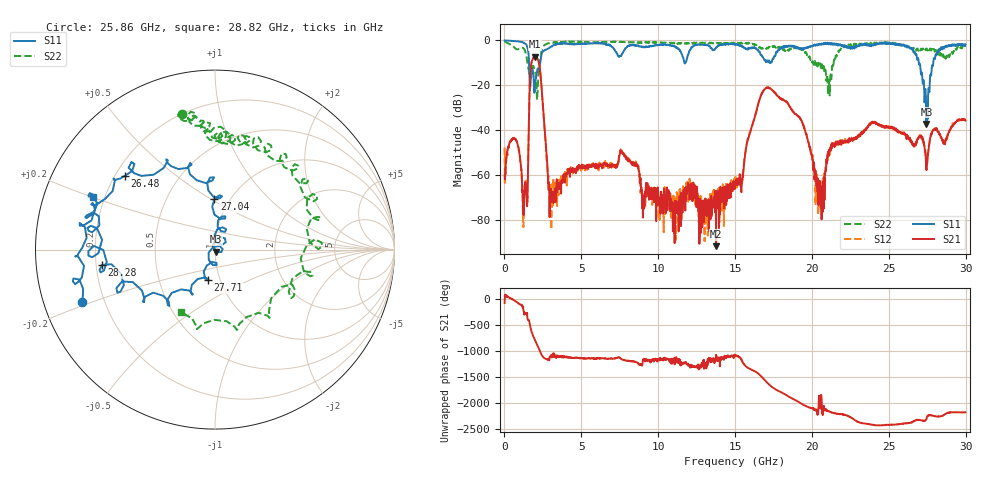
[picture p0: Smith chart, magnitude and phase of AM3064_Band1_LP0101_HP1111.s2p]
# Hz S DB R 50.0
!freq dBS11 angS11 dBS21 angS21 dBS12 angS12 dBS22 angS22
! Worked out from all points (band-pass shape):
!   1600 points, 10 MHz to 29.98 GHz, reference 50 ohm
!   highest |S21| = -7.22 dB at 1.978 GHz (marker M1); lowest = -91.4 dB at 13.77 GHz (marker M2)
!   |S21| within 3 dB of the highest: 1.748 GHz to 2.249 GHz (501.2 MHz wide, 25.1 % of centre)
!   lowest |S11| = -37.1 dB at 27.45 GHz (marker M3), VSWR 1.03, Z = 50.7 - j1.21 ohm
!   |S11| at or under -10 dB: 1.599 GHz to 2.327 GHz (728 MHz wide, 37.1 % of centre); 11.71 GHz to 11.77 GHz (61.48 MHz wide, 0.524 % of centre); 26.95 GHz to 27.89 GHz (939.6 MHz wide, 3.43 % of centre)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
!   |S22| runs from -26.4 to -0.4 dB; largest |S21 - S12| = 0.0092
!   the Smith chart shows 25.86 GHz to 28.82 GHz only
!   S11 on the Smith chart (normalised r, x): 25.86 GHz: 0.12, -0.19; 26.48 GHz: 0.24, +0.34; 27.04 GHz: 0.85, +0.52; 27.71 GHz: 0.87, -0.31; 28.28 GHz: 0.22, -0.06; 28.82 GHz: 0.16, +0.20
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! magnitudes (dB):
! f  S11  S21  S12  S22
! 10 MHz  0.0  -60.0  -47.6  -0.4
! 722.3 MHz  -0.3  -44.1  -44.0  -3.7
! 1.341 GHz  -1.4  -65.1  -65.8  -4.6
! 1.978 GHz  -20.8  -7.2  -7.2  -13.5
! 3.065 GHz  -2.6  -72.0  -74.7  -1.0
! 5.015 GHz  -1.4  -55.8  -56.5  -0.7
! 10 GHz  -2.0  -67.2  -68.2  -0.9
! 13.77 GHz  -3.2  -91.4  -66.0  -1.2
! 15 GHz  -1.8  -62.8  -63.0  -1.4
! 17.05 GHz  -9.2  -21.0  -21.0  -3.8
! 19.99 GHz  -2.8  -51.2  -51.6  -9.1
! 20.67 GHz  -1.5  -64.5  -70.5  -11.0
! 21.27 GHz  -1.3  -46.0  -46.9  -17.3
! 25 GHz  -1.0  -38.5  -38.3  -1.2
! 25.86 GHz  -2.0  -41.0  -41.4  -2.2
! 26.48 GHz  -3.8  -45.6  -44.7  -3.4
! 27.04 GHz  -11.0  -42.4  -42.0  -4.6
! 27.45 GHz  -37.1  -57.6  -54.2  -3.6
! 27.71 GHz  -15.2  -42.9  -42.2  -3.7
! 28.28 GHz  -3.9  -41.5  -41.4  -5.2
! 28.82 GHz  -2.6  -42.1  -42.4  -8.0
! 29.98 GHz  -1.8  -35.7  -34.8  -2.9
